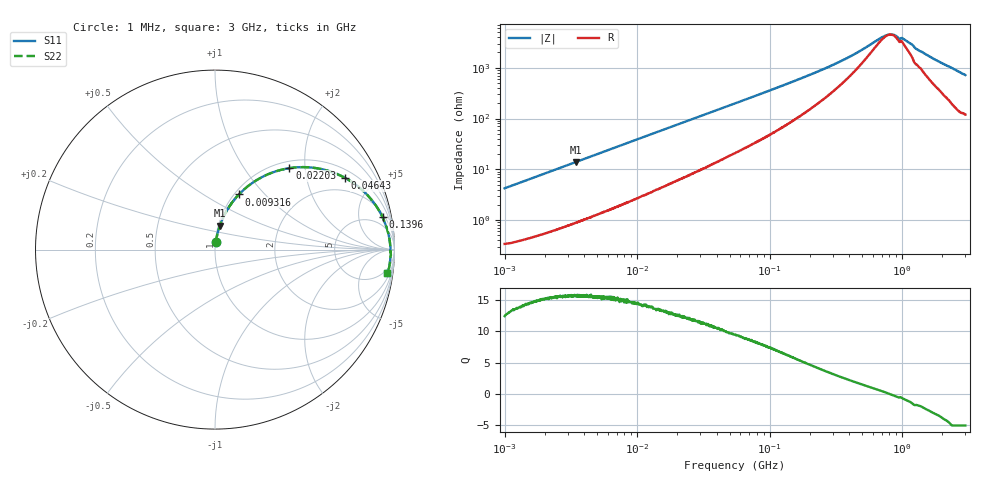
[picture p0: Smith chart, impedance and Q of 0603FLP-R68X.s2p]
!s-Parameter Generated by FASTRON Sdn. Bhd.
!FASTRON P/N : 0603FLP-R68X
!Keysight Technologies: E4991B_MY54100416_A.01.15
!Date: Tue Dec 02 12:56:09 2025
!Version  :Rev00  Tue Dec 02 12:56:09 2025
!Data & Calibration Information:
!Freq  S11  S21  S12  S22
!PortZ  Port1:50+j0  Port2:50+j0
!When reading reference impedance value at option line is always used.
! Remarks : This data is being provided solely for informational purposes.
# Hz S dB R 50
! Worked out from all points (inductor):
!   1601 points, 1 MHz to 3 GHz, reference 50 ohm
!   read as one part in series: L = 666 nH near 1.041 MHz
!   highest Q = 15.7 at 3.442 MHz (marker M1), where L = 642 nH
!   self-resonance near 810.8 MHz
!   S11 on the Smith chart (normalised r, x): 1 MHz: 1.01, +0.08; 9.316 MHz: 1.05, +0.73; 22.03 MHz: 1.13, +1.66; 46.43 MHz: 1.34, +3.37; 139.6 MHz: 3, +10; 3 GHz: 3, -14
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1000000  -27.50 83.0  -0.04 -2.4  -0.04 -2.4  -27.50 83.0
3441760  -17.30 78.5  -0.16 -7.8  -0.16 -7.8  -17.30 78.5
3804036  -16.50 77.7  -0.18 -8.6  -0.18 -8.6  -16.50 77.7
6180806  -12.60 72.7  -0.38 -13.5  -0.38 -13.5  -12.60 72.7
9316388  -9.51 66.6  -0.73 -19.5  -0.73 -19.5  -9.51 66.6
1.447069e7  -6.54 57.8  -1.43 -28.0  -1.43 -28.0  -6.54 57.8
2.20312e7  -4.22 47.6  -2.61 -37.8  -2.61 -37.8  -4.22 47.6
3.158701e7  -2.74 38.3  -4.12 -46.6  -4.12 -46.6  -2.74 38.3
4.643495e7  -1.66 29.0  -6.25 -55.3  -6.25 -55.3  -1.66 29.0
5.504702e7  -1.32 25.3  -7.33 -58.7  -7.33 -58.7  -1.32 25.3
8.422788e7  -0.76 17.5  -10.40 -65.4  -10.40 -65.4  -0.76 17.5
1.396205e8  -0.43 10.9  -14.40 -69.8  -14.40 -69.8  -0.43 10.9
2.083556e8  -0.31 7.2  -17.90 -70.4  -17.90 -70.4  -0.31 7.2
3.779341e8  -0.23 3.4  -23.90 -64.1  -23.90 -64.1  -0.23 3.4
6.889699e8  -0.20 0.7  -31.90 -27.4  -31.90 -27.4  -0.20 0.7
7.925923e8  -0.19 0.1  -33.20 -4.2  -33.20 -4.2  -0.19 0.1
8.586597e8  -0.19 -0.2  -33.20 11.2  -33.20 11.2  -0.19 -0.2
9.395906e8  -0.20 -0.7  -31.90 26.9  -31.90 26.9  -0.20 -0.7
1.023018e9  -0.19 -0.9  -31.50 36.3  -31.50 36.3  -0.19 -0.9
1.313842e9  -0.19 -2.2  -27.30 58.9  -27.30 58.9  -0.19 -2.2
1.773925e9  -0.20 -3.7  -23.40 68.7  -23.40 68.7  -0.20 -3.7
3e9  -0.28 -7.6  -17.40 72.8  -17.40 72.8  -0.28 -7.6
